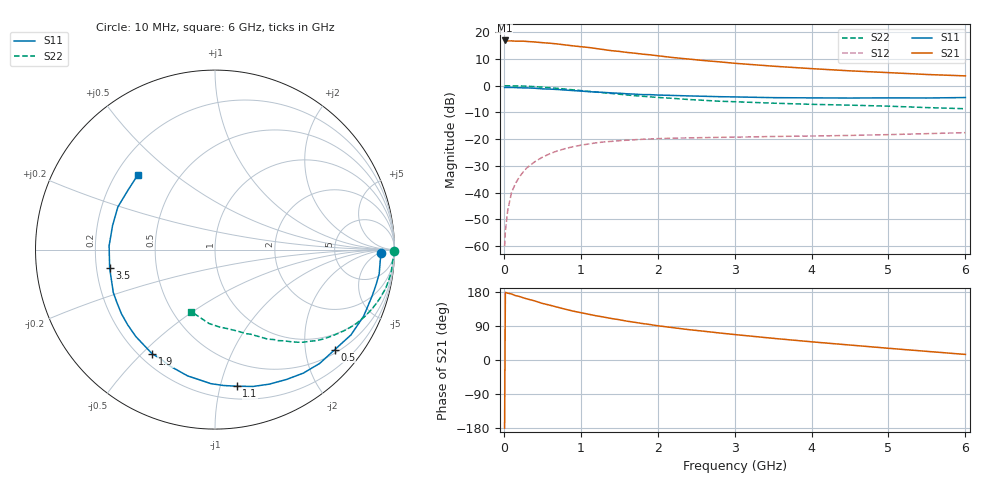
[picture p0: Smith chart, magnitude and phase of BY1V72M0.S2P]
! SIEMENS Small Signal Semiconductors
! BFY420
! Si NPN RF SIEGET Grounded Emitter Transistor in MICRO-X
! VCE = 1.75 V  IC = 2 mA
! Common Emitter S-Parameters:  October  1996
# GHz  S  MA  R  50
!  f  S11  S21  S12  S22
! GHz  MAG  ANG  MAG  ANG  MAG  ANG  MAG  ANG
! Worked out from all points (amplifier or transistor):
!   36 points, 10 MHz to 6 GHz, reference 50 ohm
!   highest |S21| = 16.9 dB at 10 MHz (marker M1)
!   |S21| within 3 dB of that: start of sweep to 1.196 GHz
!   unconditionally stable (mu >= 1): 3.987 GHz to end of sweep
!   at 250 MHz: K = 0.06, MSG = 24.5 dB, |S12| = -32.3 dB
!   at 1.4 GHz: K = 0.30, MSG = 16.9 dB, |S12| = -20.8 dB
!   at 6 GHz: K = 1.26, MAG = 7.6 dB, |S12| = -17.6 dB
!   S11 on the Smith chart (normalised r, x): 10 MHz: 23, -6; 500 MHz: 0.58, -2.64; 1.1 GHz: 0.30, -1.13; 1.9 GHz: 0.25, -0.54; 3.5 GHz: 0.25, -0.08; 6 GHz: 0.29, +0.38
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0.01  0.9225 -1.1  6.981 -179.6  0.001 97.7  0.9964 -0.4
0.02  0.9245 -1.9  6.962 178.4  0.0019 97.5  0.9929 -0.8
0.05  0.9226 -4.0  6.838 176.4  0.0046 88.7  0.9949 -2.1
0.1  0.9247 -8.4  6.852 174.2  0.0101 84.2  0.9906 -4.3
0.15  0.9186 -12.2  6.781 170.0  0.0147 83.2  0.9905 -6.4
0.2  0.9132 -16.2  6.784 167.8  0.0195 80.7  0.9868 -8.5
0.25  0.908 -20.5  6.779 164.4  0.0242 77.4  0.9806 -10.6
0.4  0.8943 -32.1  6.546 156.0  0.0376 71.8  0.9574 -16.6
0.5  0.8694 -39.9  6.347 149.4  0.0458 67.2  0.9362 -20.6
0.7  0.8461 -54.4  5.994 139.2  0.0606 59.1  0.8888 -27.7
0.8  0.8262 -61.1  5.753 134.0  0.0667 54.9  0.861 -30.9
0.9  0.8084 -68.0  5.533 129.1  0.0723 51.5  0.8343 -33.8
1.1  0.7709 -80.9  5.164 120.8  0.0811 45.5  0.783 -39.5
1.4  0.7301 -97.0  4.495 109.5  0.0908 37.9  0.7137 -46.3
1.6  0.7036 -107.4  4.174 102.5  0.0956 33.7  0.6688 -50.2
1.9  0.6783 -121.0  3.761 93.6  0.1006 28.5  0.6168 -55.3
2.2  0.6553 -132.3  3.344 85.3  0.1042 24.5  0.5782 -59.6
2.8  0.6212 -151.6  2.781 71.4  0.1079 18.9  0.5113 -67.2
3.5  0.5959 -170.1  2.309 57.2  0.1121 15.0  0.4701 -74.8
4.5  0.5862 166.9  1.889 39.5  0.1173 11.7  0.4317 -86.8
5.5  0.5873 145.2  1.614 22.8  0.1266 9.7  0.3887 -102.0
6  0.5986 135.8  1.52 14.7  0.1323 8.9  0.3699 -110.9
